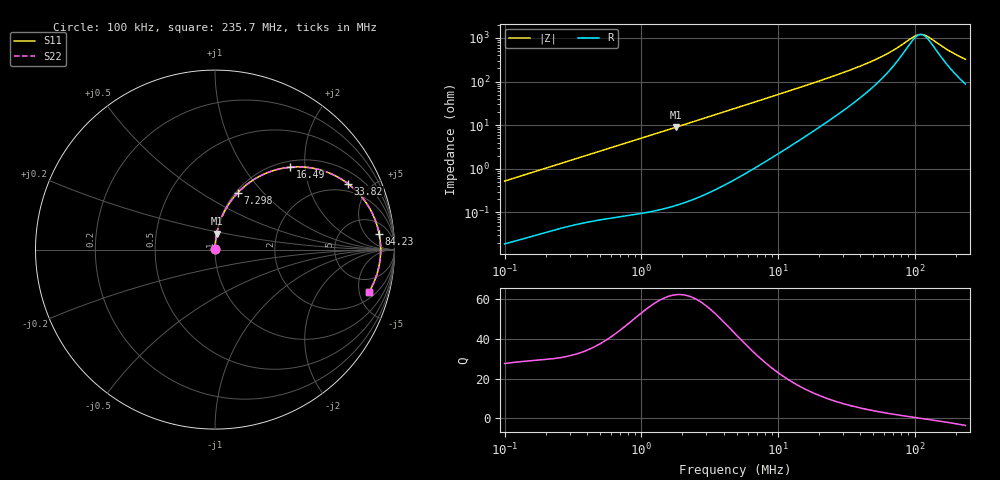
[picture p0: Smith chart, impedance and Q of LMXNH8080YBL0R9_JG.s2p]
! LMXNH8080YBL0R9_JG  S-PARAMETER MODEL  ( General Type )
! Model Generated by TAIYO YUDEN Corporation (http://www.ty-top.com)
! Version 1.0
! TAIYO YUDEN Control No. 191025NI43SB-FBB
! Copyright(c) 2019 TAIYO YUDEN CO.,LTD. All Rights Reserved.
! Product Description (link to TY-COMPAS)
! https://ds.yuden.co.jp/TYCOMPAS/or/detail?pn=LMXNH8080YBL0R9NJG&u=M
! Products Name : Inductors
! Characteristics :
!  Inductance : 0.90 uH , SRF(min) : 85 MHz , DC Resistance(max) : 0.0078 Ohm
!  Rated Current : Saturation :13000 mA , Temp Rise : 7800 mA
!  Case Size : 8.0 x 8.0 / 0.315 x 0.315 [mm/inch] , Thickness : 4.2 / 0.165 [mm/inch]
!  (Conditions: Temperature = 25 degC , DC Bias Current/Voltage = 0A / 0V)
! External Node Assignments :
!  1  o---GGG---o  2
! GND o---------o GND
! Frequency Range : 0.1MHz  -  235.669543MHz  [ 402 STEP ]
# MHz S RI R 50
! Freq[MHz].  S11 Real  S11 Imag  S21 Real  S21 Imag  S12 Real  S12 Imag  S22 Real  S22 Imag
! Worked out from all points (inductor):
!   401 points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, 100 kHz to 235.7 MHz, reference 50 ohm
!   read as one part in series: L = 827 nH near 104 kHz
!   highest Q = 62.1 at 1.804 MHz (marker M1), where L = 795 nH
!   self-resonance near 111.2 MHz
!   S11 on the Smith chart (normalised r, x): 100 kHz: 1.00, +0.01; 7.298 MHz: 1.02, +0.73; 16.49 MHz: 1.12, +1.67; 33.82 MHz: 1.56, +3.63; 84.23 MHz: 11, +12; 235.7 MHz: 2.75, -6.24
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0.1  0.000217 0.00522  0.9998 -0.00522  0.9998 -0.00522  0.000217 0.00522
0.367165  0.000909 0.0186  0.9991 -0.0186  0.9991 -0.0186  0.000909 0.0186
1.348099  0.00565 0.067  0.9944 -0.067  0.9944 -0.067  0.00565 0.067
1.803778  0.00947 0.0891  0.9905 -0.0891  0.9905 -0.0891  0.00947 0.0891
2.988015  0.0243 0.1452  0.9757 -0.1452  0.9757 -0.1452  0.0243 0.1452
4.854581  0.0604 0.2267  0.9396 -0.2267  0.9396 -0.2267  0.0604 0.2267
7.297896  0.1258 0.3157  0.8742 -0.3157  0.8742 -0.3157  0.1258 0.3157
10.76001  0.237 0.4025  0.763 -0.4025  0.763 -0.4025  0.237 0.4025
16.49262  0.419 0.4591  0.581 -0.4591  0.581 -0.4591  0.419 0.4591
17.8243  0.4565 0.4611  0.5435 -0.4611  0.5435 -0.4611  0.4565 0.4611
24.3167  0.6054 0.4382  0.3946 -0.4382  0.3946 -0.4382  0.6054 0.4382
33.8242  0.7406 0.3674  0.2594 -0.3674  0.2594 -0.3674  0.7406 0.3674
47.97127  0.8402 0.2636  0.1598 -0.2636  0.1598 -0.2636  0.8402 0.2636
65.44454  0.8926 0.1649  0.1074 -0.1649  0.1074 -0.1649  0.8926 0.1649
84.23125  0.915 0.0856  0.085 -0.0856  0.085 -0.0856  0.915 0.0856
102.2777  0.9223 0.0256  0.0777 -0.0256  0.0777 -0.0256  0.9223 0.0256
110.536  0.9231 0.00179  0.0769 -0.00179  0.0769 -0.00179  0.9231 0.00179
117.1645  0.9228 -0.0161  0.0772 0.0161  0.0772 0.0161  0.9228 -0.0161
129.107  0.9208 -0.046  0.0792 0.046  0.0792 0.046  0.9208 -0.046
183.1064  0.8963 -0.155  0.1037 0.155  0.1037 0.155  0.8963 -0.155
213.8699  0.8753 -0.2044  0.1247 0.2044  0.1247 0.2044  0.8753 -0.2044
235.6695  0.8585 -0.2354  0.1415 0.2354  0.1415 0.2354  0.8585 -0.2354
